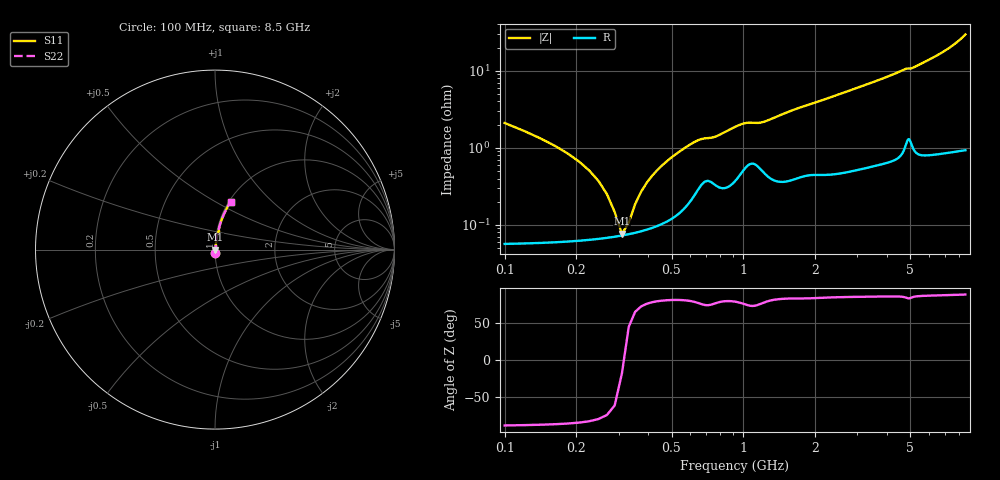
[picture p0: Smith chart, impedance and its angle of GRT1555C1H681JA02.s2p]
!Murata Part Number: GRT1555C1H681JA02
!These Parameters are Measured in Series Mode Connection
!Data Generated on Jun 19, 2026
!  o--ll--o
!Port1  Port2
!  o------o
!Operation Temp=25[degC], DC Bias Voltage=0[V]
!Freq. Start=100[MHz] Stop=9[GHz] 401[Steps]
# Hz S RI R 50
!Freq.(Hz) S11(Real) S11(Imag) S21(Real) S21(Imag) S12(Real) S12(Imag) S22(Real) S22(Imag)
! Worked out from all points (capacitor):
!   401 points, 100 MHz to 8.5 GHz, reference 50 ohm
!   read as one part in series: C = 678 pF near 142 MHz
!   lowest |Z| = 76.7 mohm at 310 MHz (marker M1)
!   series resonance near 315 MHz, so ESL is about 380 pH
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1e8  0.00101 -0.021  0.999 0.021  0.999 0.021  0.00101 -0.021
1.42e8  0.000757 -0.0131  0.9992 0.0131  0.9992 0.0131  0.000757 -0.0131
2.05e8  0.000666 -0.0066  0.9993 0.0066  0.9993 0.0066  0.000666 -0.0066
2.26e8  0.000665 -0.00505  0.9993 0.00505  0.9993 0.00505  0.000665 -0.00505
2.68e8  0.000685 -0.00243  0.9993 0.00243  0.9993 0.00243  0.000685 -0.00243
2.89e8  0.000704 -0.00129  0.9993 0.00129  0.9993 0.00129  0.000704 -0.00129
3.1e8  0.000729 -0.000237  0.9993 0.000237  0.9993 0.000237  0.000729 -0.000237
3.31e8  0.000758 0.00075  0.9992 -0.00075  0.9992 -0.00075  0.000758 0.00075
3.52e8  0.000793 0.00168  0.9992 -0.00168  0.9992 -0.00168  0.000793 0.00168
3.94e8  0.00088 0.00343  0.9991 -0.00343  0.9991 -0.00343  0.00088 0.00343
4.57e8  0.00106 0.00584  0.9989 -0.00584  0.9989 -0.00584  0.00106 0.00584
5.41e8  0.00151 0.00887  0.9985 -0.00887  0.9985 -0.00887  0.00151 0.00887
6.25e8  0.00258 0.0117  0.9974 -0.0117  0.9974 -0.0117  0.00258 0.0117
9.82e8  0.0051 0.0196  0.9949 -0.0196  0.9949 -0.0196  0.0051 0.0196
1.213e9  0.00524 0.021  0.9948 -0.021  0.9948 -0.021  0.00524 0.021
1.507e9  0.00443 0.0281  0.9956 -0.0281  0.9956 -0.0281  0.00443 0.0281
2.053e9  0.00598 0.0392  0.994 -0.0392  0.994 -0.0392  0.00598 0.0392
2.914e9  0.00835 0.0574  0.9917 -0.0574  0.9917 -0.0574  0.00835 0.0574
4.3e9  0.015 0.0894  0.985 -0.0894  0.985 -0.0894  0.015 0.0894
5.707e9  0.0239 0.1251  0.9761 -0.1251  0.9761 -0.1251  0.0239 0.1251
7.114e9  0.0423 0.1799  0.9577 -0.1799  0.9577 -0.1799  0.0423 0.1799
8.5e9  0.0878 0.2678  0.9122 -0.2678  0.9122 -0.2678  0.0878 0.2678
